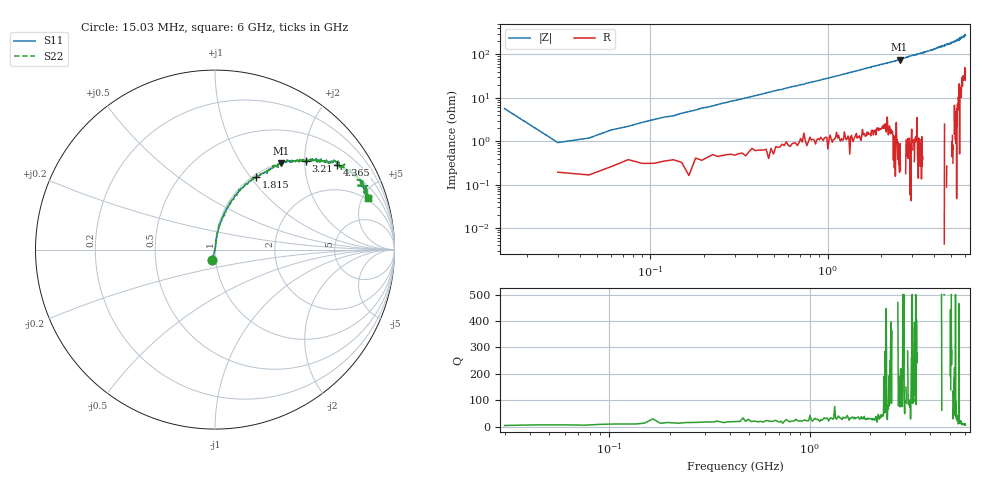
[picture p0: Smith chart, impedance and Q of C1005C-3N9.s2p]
!	Network	Analyzer	HP8753E.07.74:	Oct	30	2002	Serial	No.	JP38451487
!	Hewlett-Packard
!	7	Sep	2009	8:23:06
!	Frequency	S11	S21	S12	S22
#	HZ	S	RI	R	50
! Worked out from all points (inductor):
!   400 points, 15.03 MHz to 6 GHz, reference 50 ohm
!   read as one part in series: L = 4.62 nH near 45.03 MHz
!   highest Q = 249 at 2.55 GHz (marker M1), where L = 4.76 nH
!   S11 on the Smith chart (normalised r, x): 15.03 MHz: 0.97, -0.11; 1.815 GHz: 1.03, +1.07; 3.21 GHz: 1.02, +2.03; 4.365 GHz: 0.96, +2.91; 6 GHz: 1.81, +5.51
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1.502992e7  -0.0144 -0.0558  1.01 0.0558  1.01 0.0558  -0.0144 -0.0558
3.002985e7  0.00203 0.00908  0.998 -0.00908  0.998 -0.00908  0.00203 0.00908
4.502978e7  0.00162 0.0117  0.998 -0.0117  0.998 -0.0117  0.00162 0.0117
6.00297e7  0.00282 0.0179  0.997 -0.0179  0.997 -0.0179  0.00282 0.0179
1.050295e8  0.00416 0.0313  0.996 -0.0313  0.996 -0.0313  0.00416 0.0313
1.95029e8  0.00688 0.0574  0.993 -0.0574  0.993 -0.0574  0.00688 0.0574
2.850286e8  0.0117 0.0823  0.988 -0.0823  0.988 -0.0823  0.0117 0.0823
6.150269e8  0.0373 0.169  0.963 -0.169  0.963 -0.169  0.0373 0.169
1.020025e9  0.0853 0.26  0.915 -0.26  0.915 -0.26  0.0853 0.26
1.815021e9  0.227 0.406  0.773 -0.406  0.773 -0.406  0.227 0.406
2.01002e9  0.264 0.425  0.736 -0.425  0.736 -0.425  0.264 0.425
2.550017e9  0.368 0.481  0.632 -0.481  0.632 -0.481  0.368 0.481
3.015015e9  0.473 0.502  0.527 -0.502  0.527 -0.502  0.473 0.502
3.210014e9  0.508 0.495  0.492 -0.495  0.492 -0.495  0.508 0.495
4.00501e9  0.65 0.492  0.35 -0.492  0.35 -0.492  0.65 0.492
4.365008e9  0.682 0.472  0.318 -0.472  0.318 -0.472  0.682 0.472
5.010005e9  0.773 0.419  0.227 -0.419  0.227 -0.419  0.773 0.419
5.355003e9  0.826 0.379  0.174 -0.379  0.174 -0.379  0.826 0.379
5.535002e9  0.795 0.357  0.205 -0.357  0.205 -0.357  0.795 0.357
5.565002e9  0.85 0.356  0.15 -0.356  0.15 -0.356  0.85 0.356
5.595002e9  0.815 0.354  0.185 -0.354  0.185 -0.354  0.815 0.354
6e9  0.853 0.288  0.147 -0.288  0.147 -0.288  0.853 0.288
